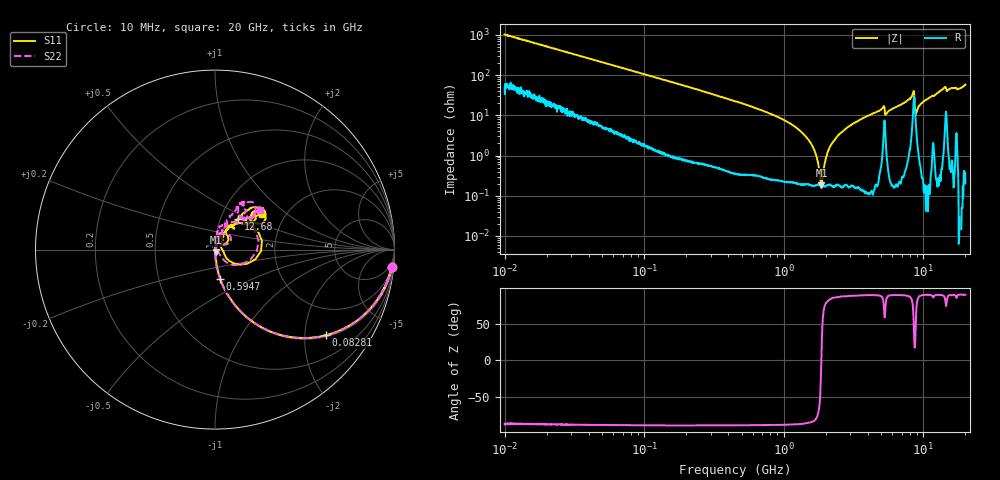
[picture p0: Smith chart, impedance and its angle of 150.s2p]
!Keysight Technologies,P5008B,MY61100088,A.16.20.02
!Date: Friday, August 30, 2024 13:38:14
!Correction: S11(C  2-Port  )
!S21(C  2-Port  )
!S12(C  2-Port  )
!S22(C  2-Port  )
!S2P File: Measurements: S11, S21, S12, S22:Log Frequency Sweep
# Hz S  MA  R 50
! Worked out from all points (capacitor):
!   1601 points, 10 MHz to 20 GHz, reference 50 ohm
!   read as one part in series: C = 15.5 pF near 10.39 MHz
!   lowest |Z| = 184 mohm at 1.86 GHz (marker M1)
!   series resonance near 1.858 GHz, so ESL is about 470 pH
!   S11 on the Smith chart (normalised r, x): 10 MHz: 2, -21; 82.81 MHz: 1.04, -2.54; 594.7 MHz: 1.00, -0.34; 12.68 GHz: 1.21, +0.44; 20 GHz: 1.53, +0.68
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1e7  0.9914 -5.5  0.09634 81.8  0.09632 81.8  0.9908 -5.5
3.555162e7  0.9383 -18.6  0.3192 69.6  0.3191 69.6  0.9381 -18.6
8.281309e7  0.7798 -37.8  0.6119 51.2  0.6116 51.1  0.7799 -37.8
1.263918e8  0.6385 -49.6  0.7602 39.5  0.7598 39.5  0.6386 -49.7
4.472136e8  0.2239 -76.5  0.9712 12.5  0.9707 12.5  0.2239 -76.9
5.947078e8  0.1656 -79.9  0.9831 8.9  0.9827 8.9  0.1654 -80.2
1.589917e9  0.03183 -85.1  0.9978 0.3  0.9974 0.2  0.032 -88.3
1.859765e9  0.01661 -75.7  0.9982 -0.9  0.9979 -1.0  0.01633 -93.1
2.035438e9  0.008095 -77.4  0.9983 -1.6  0.9981 -1.7  0.008493 -79.2
2.238313e9  0.002913 11.5  0.9985 -2.4  0.9982 -2.4  0.0006438 -6.1
2.449743e9  0.008718 86.2  0.9987 -3.1  0.9982 -3.2  0.009068 59.4
2.865525e9  0.02294 86.5  0.9984 -4.5  0.998 -4.5  0.02247 74.7
5.067356e9  0.08791 75.5  0.9882 -11.8  0.9878 -11.8  0.08974 69.1
5.652411e9  0.05944 76.4  0.9964 -11.3  0.996 -11.4  0.06263 72.6
8.384452e9  0.2174 42.5  0.9078 -24.6  0.9078 -24.7  0.207 45.3
8.961046e9  0.0509 -17.0  0.9734 -14.2  0.9733 -14.4  0.01345 -26.4
9.220141e9  0.04134 31.6  0.9918 -16.8  0.9913 -17.0  0.03171 71.0
9.995649e9  0.08599 57.5  0.9986 -20.8  0.998 -20.9  0.08426 74.4
1.267559e10  0.2146 53.5  0.9822 -29.3  0.9823 -29.6  0.2121 64.4
1.400536e10  0.3259 46.2  0.9457 -34.6  0.9457 -34.9  0.318 57.6
1.801527e10  0.2305 45.0  0.9792 -41.7  0.9789 -42.0  0.2242 50.9
2e10  0.3301 36.9  0.9464 -50.4  0.9466 -50.8  0.333 41.5
